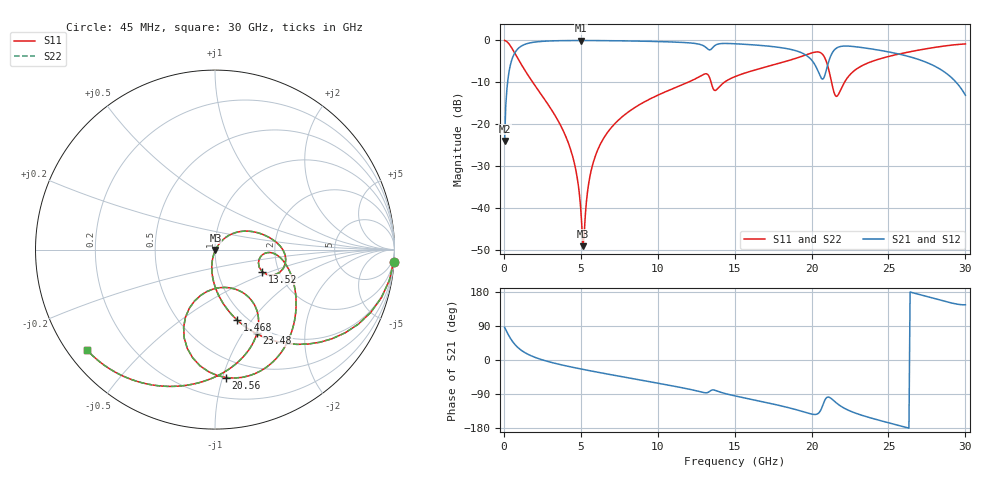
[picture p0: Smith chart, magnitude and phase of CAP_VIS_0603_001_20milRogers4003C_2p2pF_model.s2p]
! S-parameter model data by Modelithics Inc.  support@modelithics.com  813-866-6335  Tampa FL USA
! S-Parameter data specifications:
! Substrate: 20-mil Rogers 4003C, substrate thickness, H=0.508mm, Dielectric constant, Er=3.75
! PCB Mounting Pad Footprint: Pad width, PadW=0.90mm , Pad length, PadL=1.00mm , Pad gap, PadG (edge-to-edge)=1.00mm , Reference planes=3.0mm apart
! Created Wed Nov 18 13:20:34 2015
# hz S ma R 50
! 2 Port Network Data from SP1.SP block
! freq  magS11  angS11  magS21  angS21  magS12  angS12  magS22  angS22
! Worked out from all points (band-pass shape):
!   401 points, 45 MHz to 30 GHz, reference 50 ohm
!   highest |S21| = -0.03 dB at 4.988 GHz (marker M1); lowest = -24.0 dB at 45 MHz (marker M2)
!   |S21| within 3 dB of the highest: 702.1 MHz to 19.39 GHz (18.69 GHz wide, 186 % of centre); 21.34 GHz to 25.38 GHz (4.045 GHz wide, 17.3 % of centre)
!   lowest |S11| = -49.2 dB at 5.137 GHz (marker M3), VSWR 1.01, Z = 50.3 - j0.236 ohm
!   |S11| at or under -10 dB: 1.871 GHz to 11.98 GHz (10.11 GHz wide, 146 % of centre); 13.47 GHz to 14.33 GHz (868.3 MHz wide, 6.25 % of centre); 21.3 GHz to 22.14 GHz (840.6 MHz wide, 3.87 % of centre)
!   |S22| runs from -49.2 to 0.0 dB; largest |S21 - S12| = 0
!   S11 on the Smith chart (normalised r, x): 45 MHz: 1, -30; 1.468 GHz: 0.90, -0.85; 13.52 GHz: 1.64, -0.44; 20.56 GHz: 0.35, -1.03; 23.48 GHz: 0.91, -1.16; 30 GHz: 0.05, -0.34
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4.5e7  0.998 -3.8  0.06274 86.2  0.06274 86.2  0.998 -3.8
4.94325e8  0.8202 -37.2  0.5714 52.7  0.5714 52.7  0.8202 -37.2
1.467862e9  0.4095 -72.7  0.9106 17.1  0.9106 17.1  0.4095 -72.7
4.088925e9  0.06629 -103.5  0.9945 -16.0  0.9945 -16.0  0.06629 -103.5
4.688025e9  0.02741 -104.5  0.9961 -21.1  0.9961 -21.1  0.02741 -104.5
4.987575e9  0.01008 -94.8  0.9963 -23.6  0.9963 -23.6  0.01008 -94.8
5.062462e9  0.006211 -82.4  0.9963 -24.2  0.9963 -24.2  0.006211 -82.4
5.13735e9  0.003469 -42.7  0.9963 -24.8  0.9963 -24.8  0.003469 -42.7
5.661562e9  0.02729 53.7  0.9957 -28.9  0.9957 -28.9  0.02729 53.7
6.410438e9  0.06421 52.0  0.9936 -34.7  0.9936 -34.7  0.06421 52.0
1.007992e10  0.2245 26.8  0.9679 -61.7  0.9679 -61.7  0.2245 26.8
1.307542e10  0.3977 -8.0  0.8397 -86.4  0.8397 -86.4  0.3977 -8.0
1.352475e10  0.2899 -25.1  0.8009 -79.2  0.8009 -79.2  0.2899 -25.1
1.50225e10  0.3691 -7.3  0.9114 -94.8  0.9114 -94.8  0.3691 -7.3
2.003996e10  0.7105 -64.8  0.5708 -143.0  0.5708 -143.0  0.7105 -64.8
2.056418e10  0.7155 -85.1  0.3724 -134.7  0.3724 -134.7  0.7155 -85.1
2.108839e10  0.4674 -112.0  0.5382 -97.8  0.5382 -97.8  0.4674 -112.0
2.16126e10  0.2137 -83.5  0.8067 -113.3  0.8067 -113.3  0.2137 -83.5
2.348479e10  0.5196 -63.2  0.8106 -148.6  0.8106 -148.6  0.5196 -63.2
2.505742e10  0.6458 -79.4  0.7253 -166.3  0.7253 -166.3  0.6458 -79.4
2.782826e10  0.8148 -111.0  0.5107 163.8  0.5107 163.8  0.8148 -111.0
3e10  0.9067 -142.1  0.2212 145.7  0.2212 145.7  0.9067 -142.1
